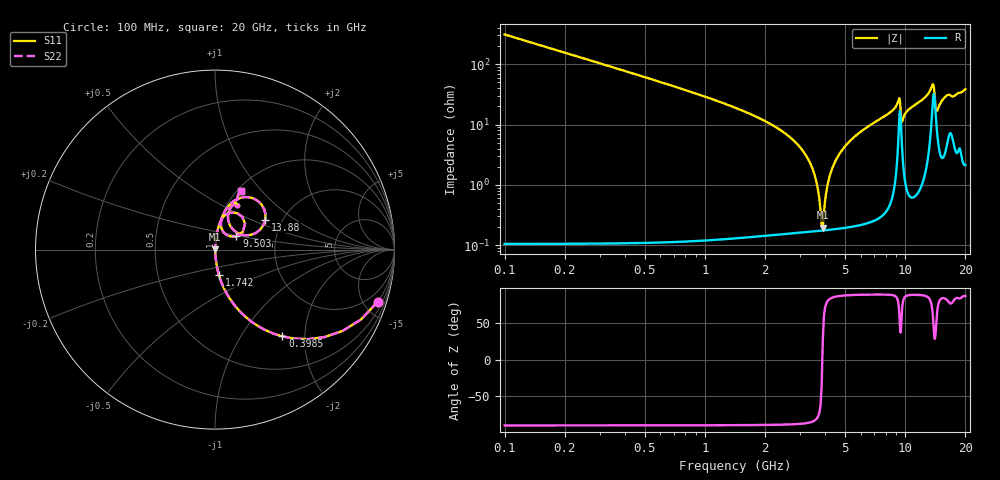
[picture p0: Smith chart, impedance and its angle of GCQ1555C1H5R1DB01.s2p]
!Murata Part Number: GCQ1555C1H5R1DB01
!These Parameters are Measured in Series Mode Connection
!Data Generated on Jan 08, 2026
!  o--ll--o
!Port1  Port2
!  o------o
!Operation Temp=25[degC], DC Bias Voltage=0[V]
!Freq. Start=100[MHz] Stop=20[GHz] 401[Steps]
# Hz S RI R 50
!Freq.(Hz) S11(Real) S11(Imag) S21(Real) S21(Imag) S12(Real) S12(Imag) S22(Real) S22(Imag)
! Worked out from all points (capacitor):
!   401 points, 100 MHz to 20 GHz, reference 50 ohm
!   read as one part in series: C = 5.1 pF near 199.5 MHz
!   lowest |Z| = 196 mohm at 3.881 GHz (marker M1)
!   series resonance near 3.86 GHz, so ESL is about 330 pH
!   S11 on the Smith chart (normalised r, x): 100 MHz: 1.00, -6.24; 398.5 MHz: 1.00, -1.55; 1.742 GHz: 1.00, -0.29; 9.503 GHz: 1.25, +0.19; 13.88 GHz: 1.64, +0.61; 20 GHz: 1.04, +0.77
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1e8  0.9067 -0.2907  0.0933 0.2907  0.0933 0.2907  0.9067 -0.2907
3.985e8  0.3753 -0.4835  0.6247 0.4835  0.6247 0.4835  0.3753 -0.4835
8.4625e8  0.1105 -0.3119  0.8895 0.3119  0.8895 0.3119  0.1105 -0.3119
1.74175e9  0.0213 -0.1396  0.9787 0.1396  0.9787 0.1396  0.0213 -0.1396
2.83625e9  0.00415 -0.0506  0.9958 0.0506  0.9958 0.0506  0.00415 -0.0506
3.43325e9  0.00205 -0.0191  0.998 0.0191  0.998 0.0191  0.00205 -0.0191
3.63225e9  0.00181 -0.0099  0.9982 0.0099  0.9982 0.0099  0.00181 -0.0099
3.7815e9  0.00175 -0.00335  0.9983 0.00335  0.9983 0.00335  0.00175 -0.00335
3.881e9  0.00175 0.00087  0.9982 -0.00087  0.9982 -0.00087  0.00175 0.00087
4.1795e9  0.00197 0.013  0.998 -0.013  0.998 -0.013  0.00197 0.013
4.62725e9  0.00276 0.0298  0.9972 -0.0298  0.9972 -0.0298  0.00276 0.0298
5.473e9  0.00549 0.0586  0.9945 -0.0586  0.9945 -0.0586  0.00549 0.0586
6.7665e9  0.0123 0.0989  0.9877 -0.0989  0.9877 -0.0989  0.0123 0.0989
9.30375e9  0.124 0.2025  0.876 -0.2025  0.876 -0.2025  0.124 0.2025
9.50275e9  0.1193 0.0745  0.8807 -0.0745  0.8807 -0.0745  0.1193 0.0745
9.652e9  0.05 0.0948  0.95 -0.0948  0.95 -0.0948  0.05 0.0948
1.005e10  0.0328 0.1481  0.9672 -0.1481  0.9672 -0.1481  0.0328 0.1481
1.338325e10  0.1637 0.2923  0.8363 -0.2923  0.8363 -0.2923  0.1637 0.2923
1.388075e10  0.2802 0.1675  0.7198 -0.1675  0.7198 -0.1675  0.2802 0.1675
1.43285e10  0.1057 0.1067  0.8943 -0.1067  0.8943 -0.1067  0.1057 0.1067
1.67165e10  0.1346 0.2434  0.8654 -0.2434  0.8654 -0.2434  0.1346 0.2434
2e10  0.1436 0.3239  0.8564 -0.3239  0.8564 -0.3239  0.1436 0.3239
